(* Logix 5000 AddOnInstructionDefinition export SPEL_Above; software revision 30.01; part 2 of 9 *)

ADD_ON_INSTRUCTION SPEL_BaseGet   (* revision 1.0, vendor SEIKO EPSON CORP. *)
// Gets the base coordinate system.
VAR_INPUT
   Start : BOOL; {required}
END_VAR
VAR_OUTPUT
   InCycle : BOOL; {access Read Only, visible}
   Done : BOOL; {access Read Only, visible}
   Error : BOOL; {access Read Only, visible}
END_VAR
VAR_INPUT
   NumAxes : INT; {required}
END_VAR
VAR_OUTPUT
   BaseX : REAL; {visible}
   BaseY : REAL; {visible}
   BaseZ : REAL; {visible}
   BaseU : REAL; {visible}
   BaseV : REAL; {visible}
   BaseW : REAL; {visible}
END_VAR
VAR_IN_OUT
   ExtInputs : AB:ETHERNET_MODULE_INT_128Bytes:I:0; {required}
   ExtOutputs : AB:ETHERNET_MODULE_INT_128Bytes:O:0; {required}
END_VAR
VAR_OUTPUT
   ErrCode1 : INT; {access Read Only, visible}
   ErrCode2 : INT; {access Read Only, visible}
END_VAR
VAR
   Coordinatex1000 : DINT; {access None}
   Coordinate_INTS : INT[2]; {access None}
   OneShotStart : BOOL[32]; {access None}
   StartInit : BOOL[32]; {access None}
   ExecBaseGetW : SPEL_ExecCmd := (MaxTime := 3000); {access None}
   ExecBaseGetV : SPEL_ExecCmd := (MaxTime := 3000); {access None}
   ExecBaseGetU : SPEL_ExecCmd := (MaxTime := 3000); {access None}
   ExecBaseGetZ : SPEL_ExecCmd := (MaxTime := 3000); {access None}
   ExecBaseGetY : SPEL_ExecCmd := (MaxTime := 3000); {access None}
   ExecBaseGetX : SPEL_ExecCmd := (MaxTime := 3000); {access None}
   X6 : BOOL; {access None}
   ExecTimeout : DINT := 5000; {access None}
END_VAR

ROUTINE Logic   (* ladder *)
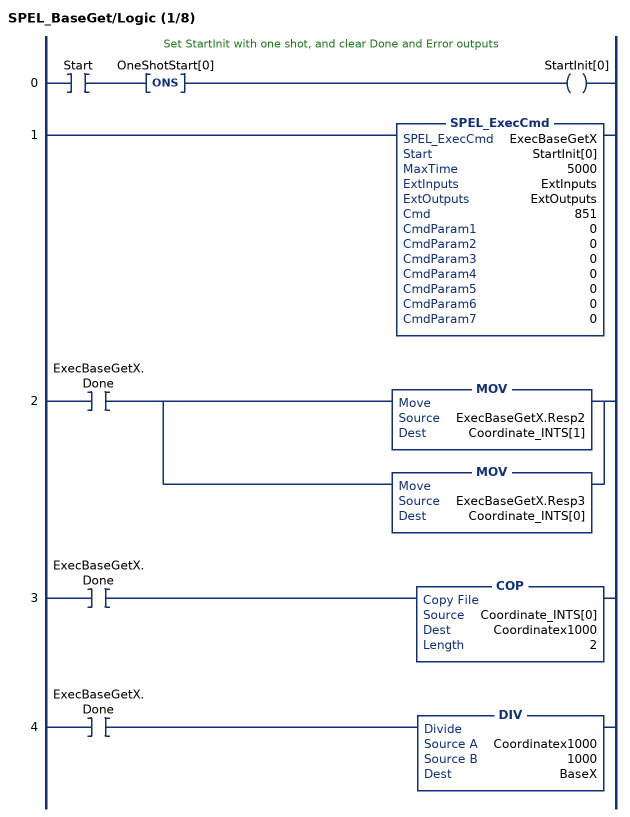
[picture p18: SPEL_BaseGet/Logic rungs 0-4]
   // Set StartInit with one shot, and clear Done and Error outputs
   0: XIC(Start)ONS(OneShotStart[0])OTE(StartInit[0]);
   1: SPEL_ExecCmd(ExecBaseGetX,StartInit[0],5000,ExtInputs,ExtOutputs,851,0,0,0,0,0,0,0);
   2: XIC(ExecBaseGetX.Done)[MOV(ExecBaseGetX.Resp2,Coordinate_INTS[1]) ,MOV(ExecBaseGetX.Resp3,Coordinate_INTS[0]) ];
   3: XIC(ExecBaseGetX.Done)COP(Coordinate_INTS[0],Coordinatex1000,2);
   4: XIC(ExecBaseGetX.Done)DIV(Coordinatex1000,1000,BaseX);
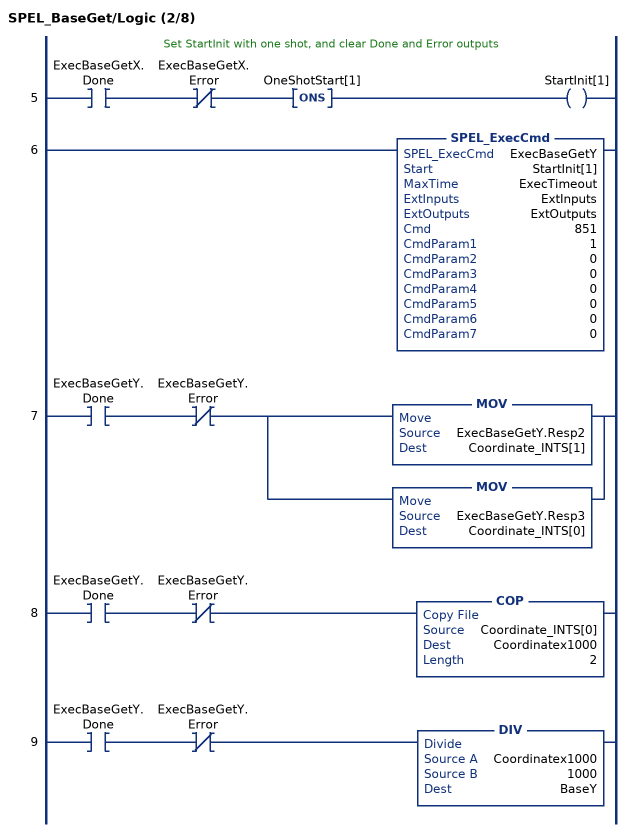
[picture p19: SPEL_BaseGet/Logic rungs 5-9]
   // Set StartInit with one shot, and clear Done and Error outputs
   5: XIC(ExecBaseGetX.Done)XIO(ExecBaseGetX.Error)ONS(OneShotStart[1])OTE(StartInit[1]);
   6: SPEL_ExecCmd(ExecBaseGetY,StartInit[1],ExecTimeout,ExtInputs,ExtOutputs,851,1,0,0,0,0,0,0);
   7: XIC(ExecBaseGetY.Done)XIO(ExecBaseGetY.Error)[MOV(ExecBaseGetY.Resp2,Coordinate_INTS[1]) ,MOV(ExecBaseGetY.Resp3,Coordinate_INTS[0]) ];
   8: XIC(ExecBaseGetY.Done)XIO(ExecBaseGetY.Error)COP(Coordinate_INTS[0],Coordinatex1000,2);
   9: XIC(ExecBaseGetY.Done)XIO(ExecBaseGetY.Error)DIV(Coordinatex1000,1000,BaseY);
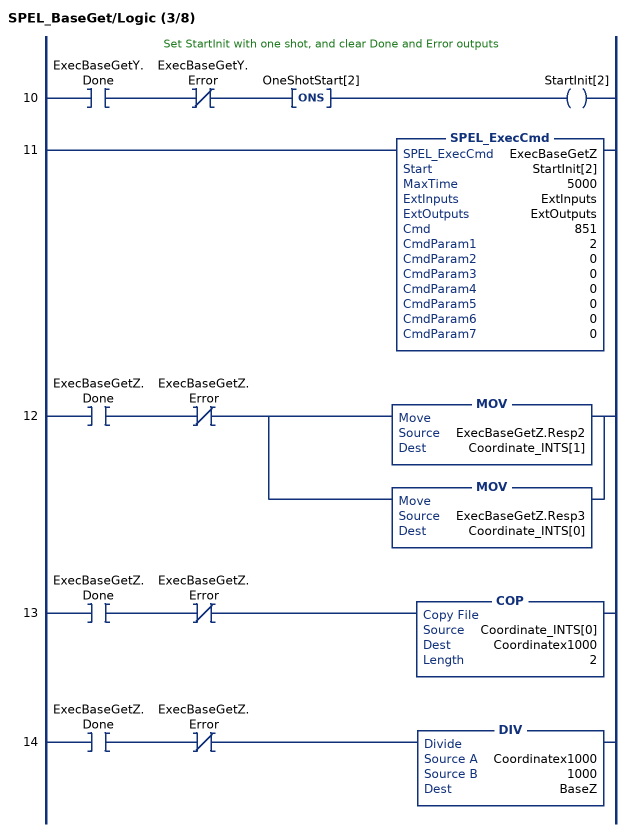
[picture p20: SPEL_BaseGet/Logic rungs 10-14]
   // Set StartInit with one shot, and clear Done and Error outputs
   10: XIC(ExecBaseGetY.Done)XIO(ExecBaseGetY.Error)ONS(OneShotStart[2])OTE(StartInit[2]);
   11: SPEL_ExecCmd(ExecBaseGetZ,StartInit[2],5000,ExtInputs,ExtOutputs,851,2,0,0,0,0,0,0);
   12: XIC(ExecBaseGetZ.Done)XIO(ExecBaseGetZ.Error)[MOV(ExecBaseGetZ.Resp2,Coordinate_INTS[1]) ,MOV(ExecBaseGetZ.Resp3,Coordinate_INTS[0]) ];
   13: XIC(ExecBaseGetZ.Done)XIO(ExecBaseGetZ.Error)COP(Coordinate_INTS[0],Coordinatex1000,2);
   14: XIC(ExecBaseGetZ.Done)XIO(ExecBaseGetZ.Error)DIV(Coordinatex1000,1000,BaseZ);
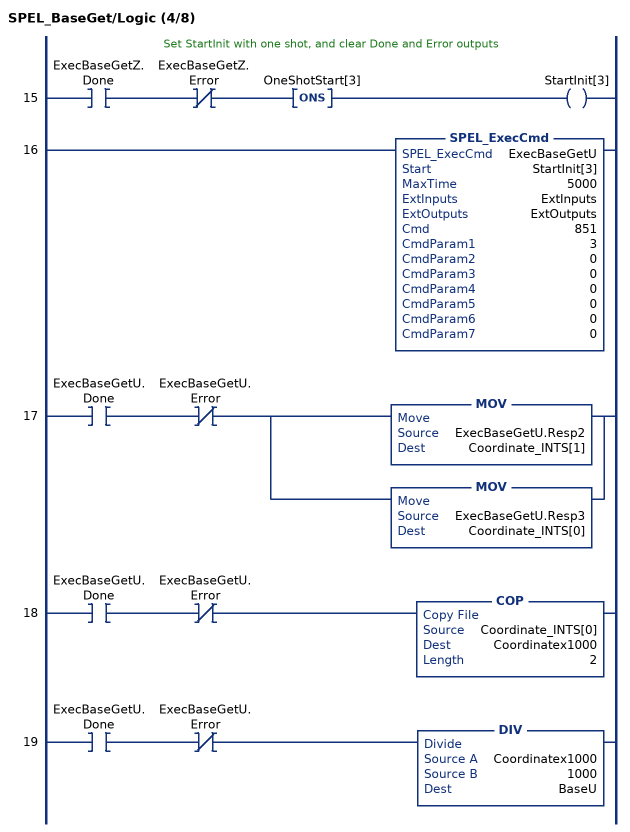
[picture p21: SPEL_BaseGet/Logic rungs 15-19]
   // Set StartInit with one shot, and clear Done and Error outputs
   15: XIC(ExecBaseGetZ.Done)XIO(ExecBaseGetZ.Error)ONS(OneShotStart[3])OTE(StartInit[3]);
   16: SPEL_ExecCmd(ExecBaseGetU,StartInit[3],5000,ExtInputs,ExtOutputs,851,3,0,0,0,0,0,0);
   17: XIC(ExecBaseGetU.Done)XIO(ExecBaseGetU.Error)[MOV(ExecBaseGetU.Resp2,Coordinate_INTS[1]) ,MOV(ExecBaseGetU.Resp3,Coordinate_INTS[0]) ];
   18: XIC(ExecBaseGetU.Done)XIO(ExecBaseGetU.Error)COP(Coordinate_INTS[0],Coordinatex1000,2);
   19: XIC(ExecBaseGetU.Done)XIO(ExecBaseGetU.Error)DIV(Coordinatex1000,1000,BaseU);
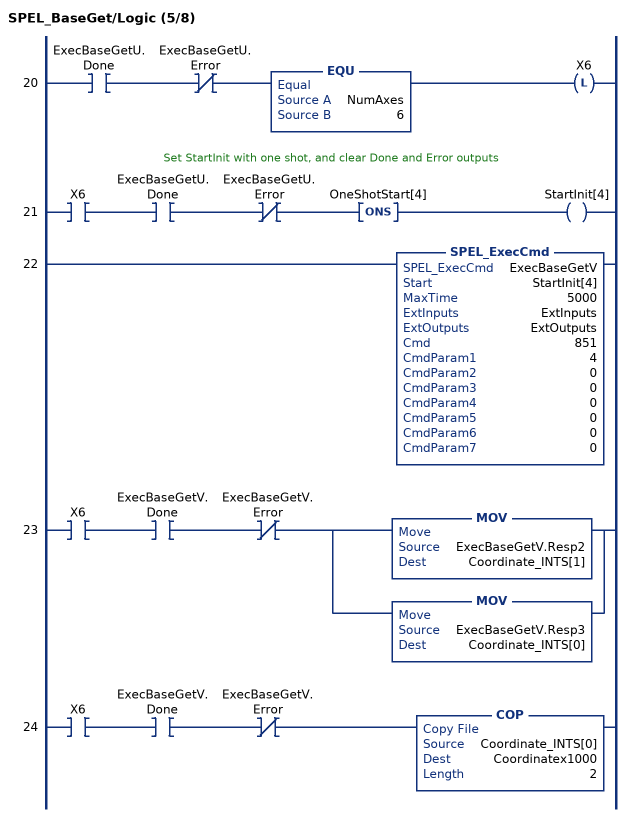
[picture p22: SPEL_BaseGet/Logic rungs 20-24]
   20: XIC(ExecBaseGetU.Done)XIO(ExecBaseGetU.Error)EQU(NumAxes,6)OTL(X6);
   // Set StartInit with one shot, and clear Done and Error outputs
   21: XIC(X6)XIC(ExecBaseGetU.Done)XIO(ExecBaseGetU.Error)ONS(OneShotStart[4])OTE(StartInit[4]);
   22: SPEL_ExecCmd(ExecBaseGetV,StartInit[4],5000,ExtInputs,ExtOutputs,851,4,0,0,0,0,0,0);
   23: XIC(X6)XIC(ExecBaseGetV.Done)XIO(ExecBaseGetV.Error)[MOV(ExecBaseGetV.Resp2,Coordinate_INTS[1]) ,MOV(ExecBaseGetV.Resp3,Coordinate_INTS[0]) ];
   24: XIC(X6)XIC(ExecBaseGetV.Done)XIO(ExecBaseGetV.Error)COP(Coordinate_INTS[0],Coordinatex1000,2);
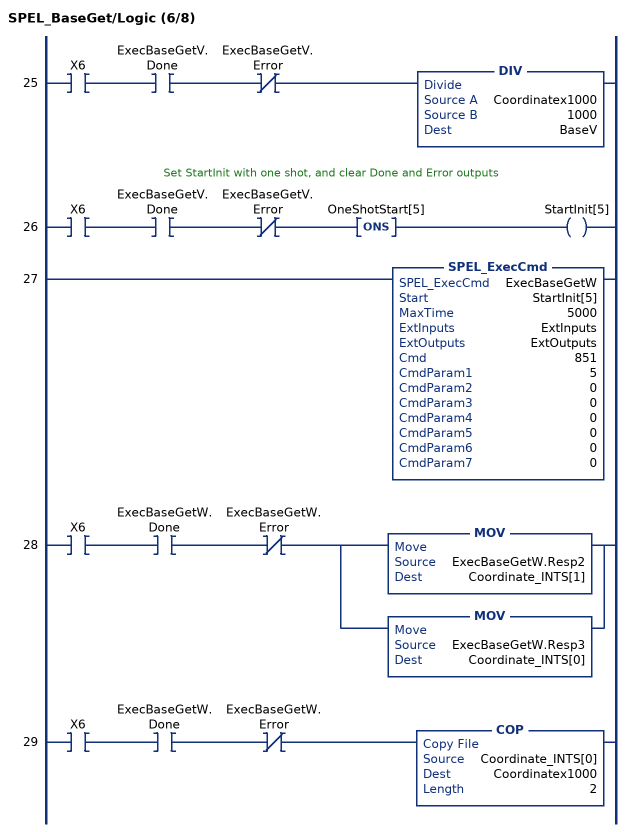
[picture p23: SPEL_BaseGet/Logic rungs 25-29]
   25: XIC(X6)XIC(ExecBaseGetV.Done)XIO(ExecBaseGetV.Error)DIV(Coordinatex1000,1000,BaseV);
   // Set StartInit with one shot, and clear Done and Error outputs
   26: XIC(X6)XIC(ExecBaseGetV.Done)XIO(ExecBaseGetV.Error)ONS(OneShotStart[5])OTE(StartInit[5]);
   27: SPEL_ExecCmd(ExecBaseGetW,StartInit[5],5000,ExtInputs,ExtOutputs,851,5,0,0,0,0,0,0);
   28: XIC(X6)XIC(ExecBaseGetW.Done)XIO(ExecBaseGetW.Error)[MOV(ExecBaseGetW.Resp2,Coordinate_INTS[1]) ,MOV(ExecBaseGetW.Resp3,Coordinate_INTS[0]) ];
   29: XIC(X6)XIC(ExecBaseGetW.Done)XIO(ExecBaseGetW.Error)COP(Coordinate_INTS[0],Coordinatex1000,2);
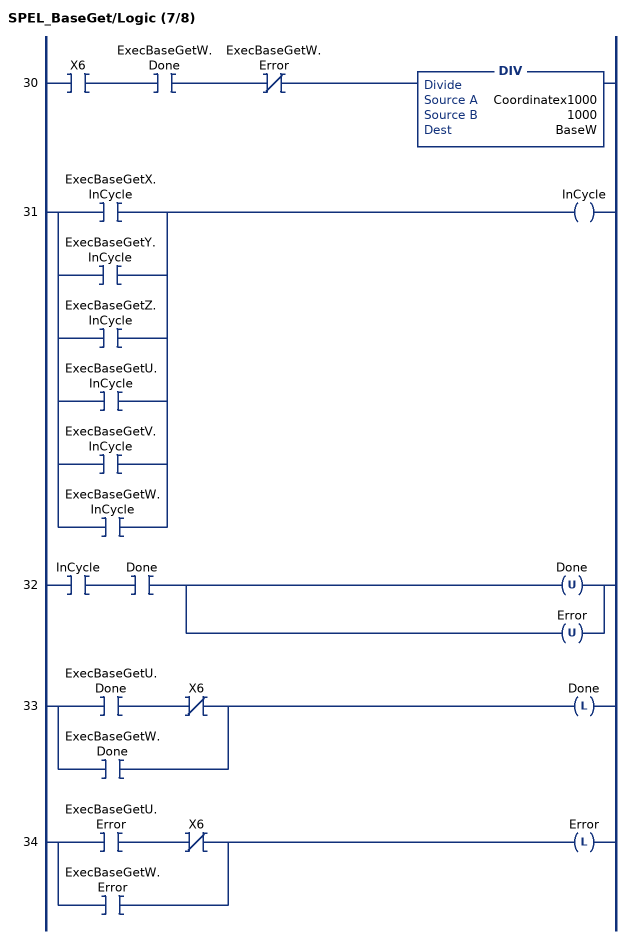
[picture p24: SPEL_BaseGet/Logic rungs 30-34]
   30: XIC(X6)XIC(ExecBaseGetW.Done)XIO(ExecBaseGetW.Error)DIV(Coordinatex1000,1000,BaseW);
   31: [XIC(ExecBaseGetX.InCycle) ,XIC(ExecBaseGetY.InCycle) ,XIC(ExecBaseGetZ.InCycle) ,XIC(ExecBaseGetU.InCycle) ,XIC(ExecBaseGetV.InCycle) ,XIC(ExecBaseGetW.InCycle) ]OTE(InCycle);
   32: XIC(InCycle)XIC(Done)[OTU(Done) ,OTU(Error) ];
   33: [XIC(ExecBaseGetU.Done) XIO(X6) ,XIC(ExecBaseGetW.Done) ]OTL(Done);
   34: [XIC(ExecBaseGetU.Error) XIO(X6) ,XIC(ExecBaseGetW.Error) ]OTL(Error);
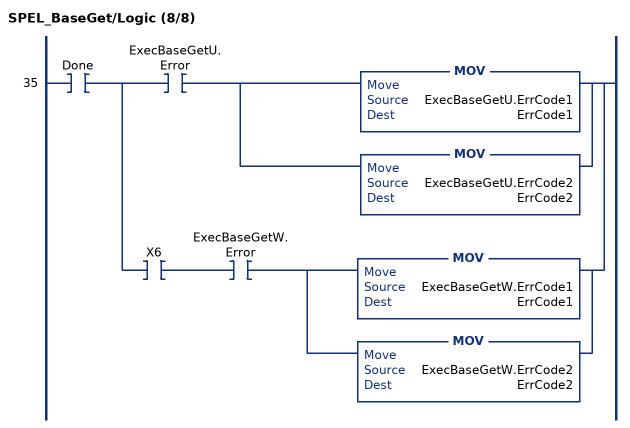
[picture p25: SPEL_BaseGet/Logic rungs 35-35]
   35: XIC(Done)[XIC(ExecBaseGetU.Error) [MOV(ExecBaseGetU.ErrCode1,ErrCode1) ,MOV(ExecBaseGetU.ErrCode2,ErrCode2) ] ,XIC(X6) XIC(ExecBaseGetW.Error) [MOV(ExecBaseGetW.ErrCode1,ErrCode1) ,MOV(ExecBaseGetW.ErrCode2,ErrCode2) ] ];
END_ROUTINE
END_ADD_ON_INSTRUCTION

ADD_ON_INSTRUCTION SPEL_BaseSet   (* revision 1.0, vendor SEIKO EPSON CORP. *)
// Sets the base coordinate system.
VAR_OUTPUT
   InCycle : BOOL; {access Read Only, visible}
   Done : BOOL; {access Read Only, visible}
END_VAR
VAR_INPUT
   Start : BOOL; {required}
END_VAR
VAR_OUTPUT
   Error : BOOL; {access Read Only, visible}
END_VAR
VAR_INPUT
   NumAxes : INT; {required}
   BaseX : REAL; {required}
   BaseY : REAL; {required}
   BaseZ : REAL; {required}
   BaseU : REAL; {required}
   BaseV : REAL; {required}
   BaseW : REAL; {required}
END_VAR
VAR_IN_OUT
   ExtInputs : AB:ETHERNET_MODULE_INT_128Bytes:I:0; {required}
   ExtOutputs : AB:ETHERNET_MODULE_INT_128Bytes:O:0; {required}
END_VAR
VAR_OUTPUT
   ErrCode1 : INT; {access Read Only, visible}
   ErrCode2 : INT; {access Read Only, visible}
END_VAR
VAR
   Valuex1000 : DINT; {access None}
   Value_INTS : INT[2]; {access None}
   StartInit : BOOL[32]; {access None}
   OneShotStart : BOOL[32]; {access None}
   ExecBaseSetX : SPEL_ExecCmd := (MaxTime := 3000); {access None}
   ExecBaseSetW : SPEL_ExecCmd := (MaxTime := 3000); {access None}
   ExecBaseSetV : SPEL_ExecCmd := (MaxTime := 3000); {access None}
   ExecBaseSetU : SPEL_ExecCmd := (MaxTime := 3000); {access None}
   ExecBaseSetZ : SPEL_ExecCmd := (MaxTime := 3000); {access None}
   ExecBaseSetY : SPEL_ExecCmd := (MaxTime := 3000); {access None}
   X6 : BOOL; {access None}
   ExecTimeout : DINT; {access None}
END_VAR

ROUTINE Logic   (* ladder *)
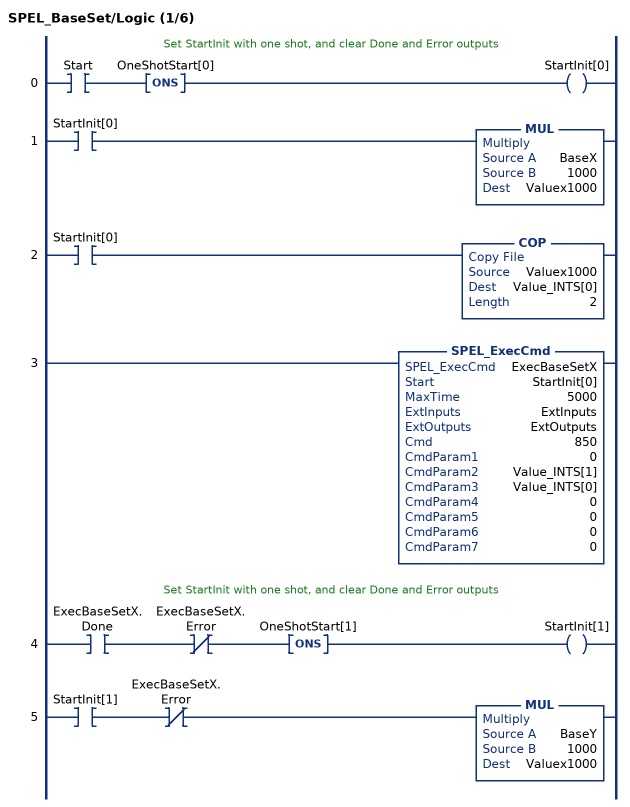
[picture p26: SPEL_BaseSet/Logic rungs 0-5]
   // Set StartInit with one shot, and clear Done and Error outputs
   0: XIC(Start)ONS(OneShotStart[0])OTE(StartInit[0]);
   1: XIC(StartInit[0])MUL(BaseX,1000,Valuex1000);
   2: XIC(StartInit[0])COP(Valuex1000,Value_INTS[0],2);
   3: SPEL_ExecCmd(ExecBaseSetX,StartInit[0],5000,ExtInputs,ExtOutputs,850,0,Value_INTS[1],Value_INTS[0],0,0,0,0);
   // Set StartInit with one shot, and clear Done and Error outputs
   4: XIC(ExecBaseSetX.Done)XIO(ExecBaseSetX.Error)ONS(OneShotStart[1])OTE(StartInit[1]);
   5: XIC(StartInit[1])XIO(ExecBaseSetX.Error)MUL(BaseY,1000,Valuex1000);
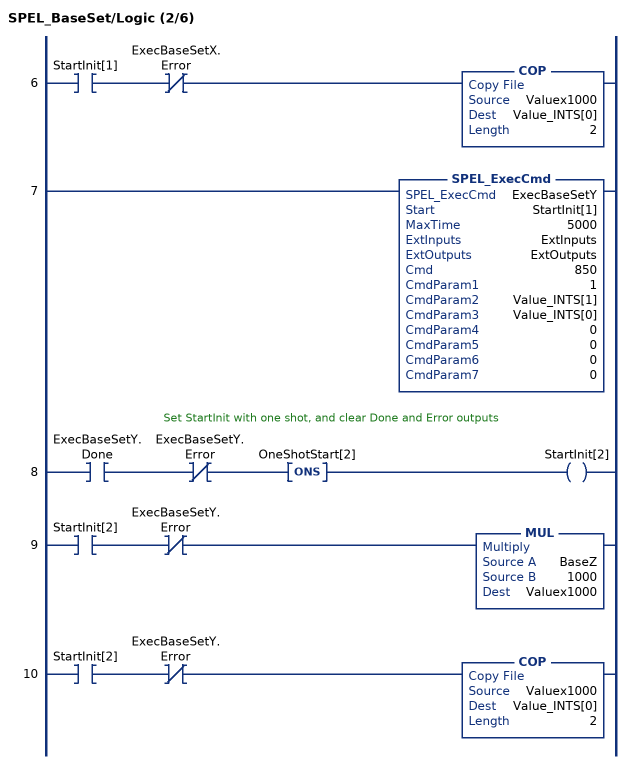
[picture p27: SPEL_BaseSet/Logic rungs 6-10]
   6: XIC(StartInit[1])XIO(ExecBaseSetX.Error)COP(Valuex1000,Value_INTS[0],2);
   7: SPEL_ExecCmd(ExecBaseSetY,StartInit[1],5000,ExtInputs,ExtOutputs,850,1,Value_INTS[1],Value_INTS[0],0,0,0,0);
   // Set StartInit with one shot, and clear Done and Error outputs
   8: XIC(ExecBaseSetY.Done)XIO(ExecBaseSetY.Error)ONS(OneShotStart[2])OTE(StartInit[2]);
   9: XIC(StartInit[2])XIO(ExecBaseSetY.Error)MUL(BaseZ,1000,Valuex1000);
   10: XIC(StartInit[2])XIO(ExecBaseSetY.Error)COP(Valuex1000,Value_INTS[0],2);
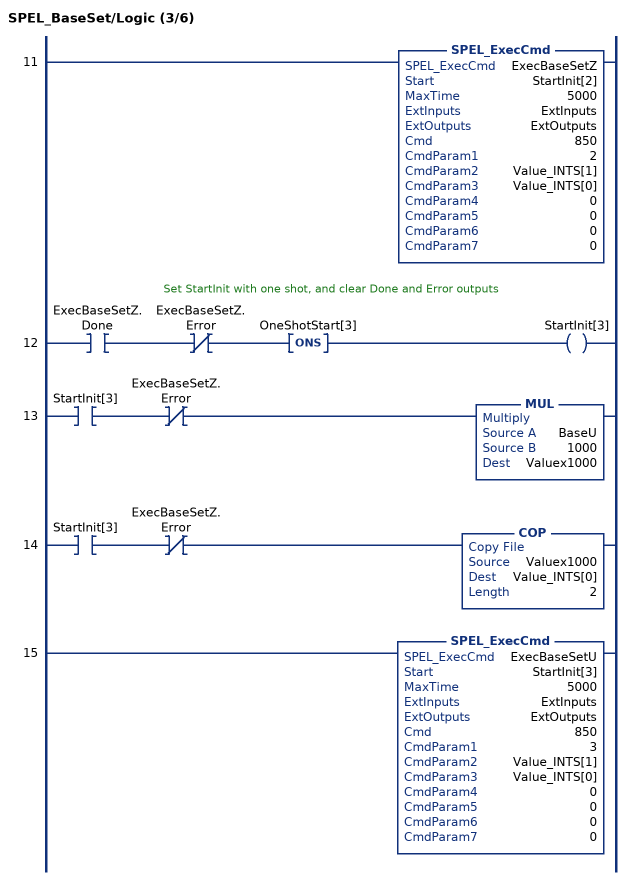
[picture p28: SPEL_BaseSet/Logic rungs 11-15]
   11: SPEL_ExecCmd(ExecBaseSetZ,StartInit[2],5000,ExtInputs,ExtOutputs,850,2,Value_INTS[1],Value_INTS[0],0,0,0,0);
   // Set StartInit with one shot, and clear Done and Error outputs
   12: XIC(ExecBaseSetZ.Done)XIO(ExecBaseSetZ.Error)ONS(OneShotStart[3])OTE(StartInit[3]);
   13: XIC(StartInit[3])XIO(ExecBaseSetZ.Error)MUL(BaseU,1000,Valuex1000);
   14: XIC(StartInit[3])XIO(ExecBaseSetZ.Error)COP(Valuex1000,Value_INTS[0],2);
   15: SPEL_ExecCmd(ExecBaseSetU,StartInit[3],5000,ExtInputs,ExtOutputs,850,3,Value_INTS[1],Value_INTS[0],0,0,0,0);
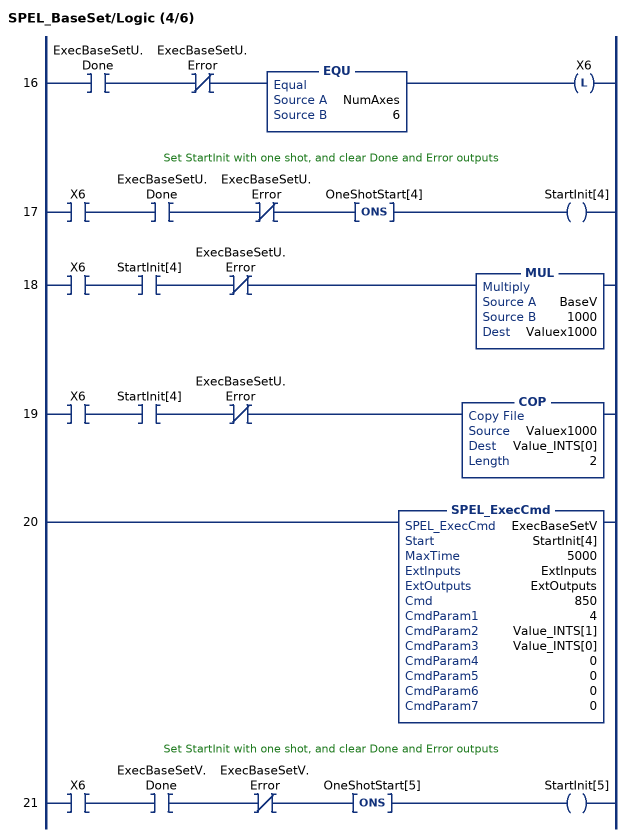
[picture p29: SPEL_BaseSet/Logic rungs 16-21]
   16: XIC(ExecBaseSetU.Done)XIO(ExecBaseSetU.Error)EQU(NumAxes,6)OTL(X6);
   // Set StartInit with one shot, and clear Done and Error outputs
   17: XIC(X6)XIC(ExecBaseSetU.Done)XIO(ExecBaseSetU.Error)ONS(OneShotStart[4])OTE(StartInit[4]);
   18: XIC(X6)XIC(StartInit[4])XIO(ExecBaseSetU.Error)MUL(BaseV,1000,Valuex1000);
   19: XIC(X6)XIC(StartInit[4])XIO(ExecBaseSetU.Error)COP(Valuex1000,Value_INTS[0],2);
   20: SPEL_ExecCmd(ExecBaseSetV,StartInit[4],5000,ExtInputs,ExtOutputs,850,4,Value_INTS[1],Value_INTS[0],0,0,0,0);
   // Set StartInit with one shot, and clear Done and Error outputs
   21: XIC(X6)XIC(ExecBaseSetV.Done)XIO(ExecBaseSetV.Error)ONS(OneShotStart[5])OTE(StartInit[5]);
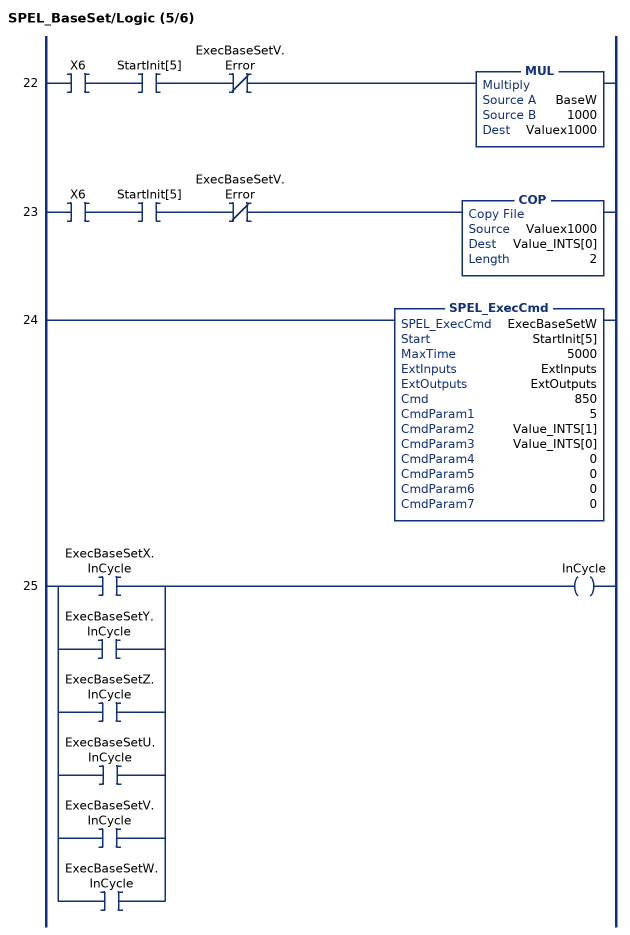
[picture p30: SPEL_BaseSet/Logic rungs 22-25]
   22: XIC(X6)XIC(StartInit[5])XIO(ExecBaseSetV.Error)MUL(BaseW,1000,Valuex1000);
   23: XIC(X6)XIC(StartInit[5])XIO(ExecBaseSetV.Error)COP(Valuex1000,Value_INTS[0],2);
   24: SPEL_ExecCmd(ExecBaseSetW,StartInit[5],5000,ExtInputs,ExtOutputs,850,5,Value_INTS[1],Value_INTS[0],0,0,0,0);
   25: [XIC(ExecBaseSetX.InCycle) ,XIC(ExecBaseSetY.InCycle) ,XIC(ExecBaseSetZ.InCycle) ,XIC(ExecBaseSetU.InCycle) ,XIC(ExecBaseSetV.InCycle) ,XIC(ExecBaseSetW.InCycle) ]OTE(InCycle);
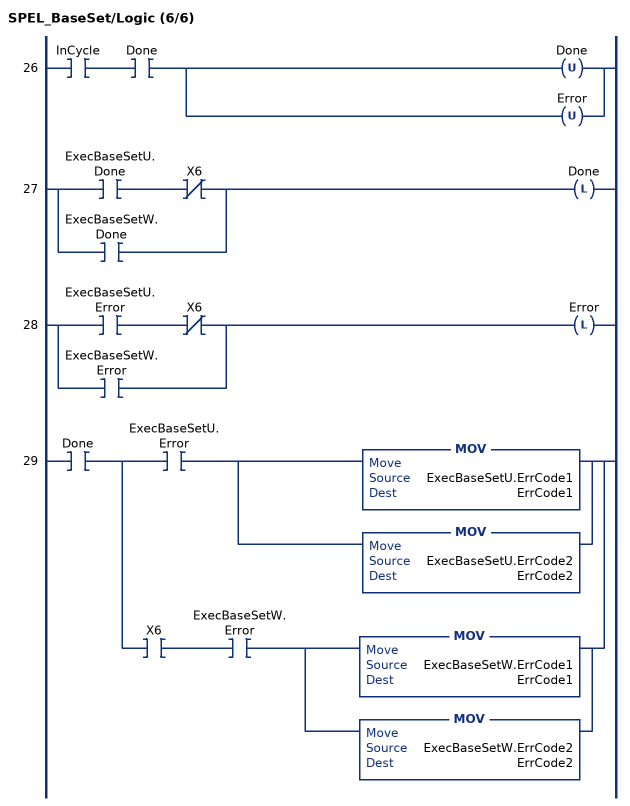
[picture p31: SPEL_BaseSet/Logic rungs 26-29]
   26: XIC(InCycle)XIC(Done)[OTU(Done) ,OTU(Error) ];
   27: [XIC(ExecBaseSetU.Done) XIO(X6) ,XIC(ExecBaseSetW.Done) ]OTL(Done);
   28: [XIC(ExecBaseSetU.Error) XIO(X6) ,XIC(ExecBaseSetW.Error) ]OTL(Error);
   29: XIC(Done)[XIC(ExecBaseSetU.Error) [MOV(ExecBaseSetU.ErrCode1,ErrCode1) ,MOV(ExecBaseSetU.ErrCode2,ErrCode2) ] ,XIC(X6) XIC(ExecBaseSetW.Error) [MOV(ExecBaseSetW.ErrCode1,ErrCode1) ,MOV(ExecBaseSetW.ErrCode2,ErrCode2) ] ];
END_ROUTINE
END_ADD_ON_INSTRUCTION

ADD_ON_INSTRUCTION SPEL_Below   (* revision 1.0, vendor SEIKO EPSON CORP. *)
// Sets the elbow orientation of the specified point to Below.
VAR_INPUT
   Start : BOOL; {required}
END_VAR
VAR_OUTPUT
   InCycle : BOOL; {access Read Only, visible}
   Done : BOOL; {access Read Only, visible}
   Error : BOOL; {access Read Only, visible}
END_VAR
VAR_INPUT
   Point : INT; {required}
END_VAR
VAR_IN_OUT
   ExtInputs : AB:ETHERNET_MODULE_INT_128Bytes:I:0; {required}
   ExtOutputs : AB:ETHERNET_MODULE_INT_128Bytes:O:0; {required}
END_VAR
VAR_OUTPUT
   ErrCode1 : INT; {access Read Only, visible}
   ErrCode2 : INT; {access Read Only, visible}
END_VAR
VAR
   ExecBelow : SPEL_ExecCmd := (MaxTime := 3000); {access None}
   OneShotStart : BOOL; {access None}
   StartCoil : BOOL; {access None}
   ExecTimeout : DINT; {access None}
END_VAR

ROUTINE Logic   (* ladder *)
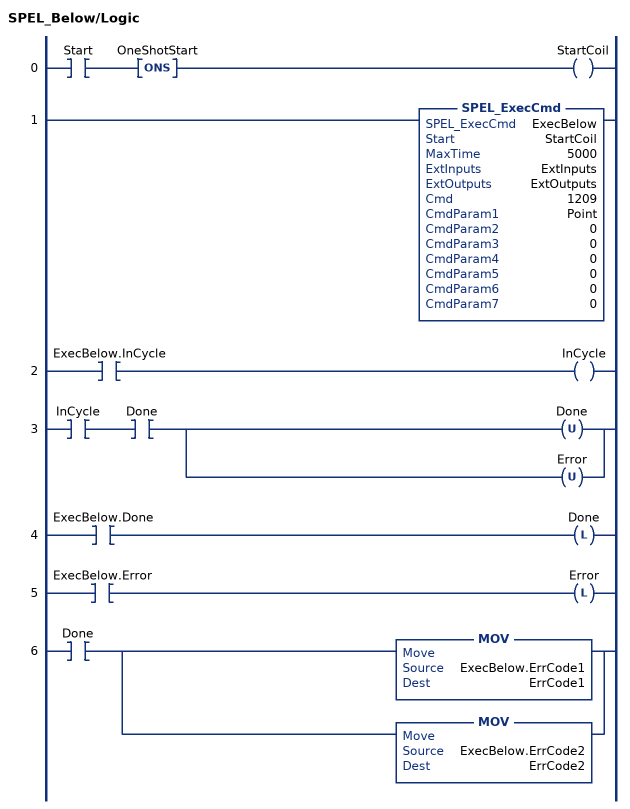
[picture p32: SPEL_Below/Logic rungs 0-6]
   0: XIC(Start)ONS(OneShotStart)OTE(StartCoil);
   1: SPEL_ExecCmd(ExecBelow,StartCoil,5000,ExtInputs,ExtOutputs,1209,Point,0,0,0,0,0,0);
   2: XIC(ExecBelow.InCycle)OTE(InCycle);
   3: XIC(InCycle)XIC(Done)[OTU(Done) ,OTU(Error) ];
   4: XIC(ExecBelow.Done)OTL(Done);
   5: XIC(ExecBelow.Error)OTL(Error);
   6: XIC(Done)[MOV(ExecBelow.ErrCode1,ErrCode1) ,MOV(ExecBelow.ErrCode2,ErrCode2) ];
END_ROUTINE
END_ADD_ON_INSTRUCTION

ADD_ON_INSTRUCTION SPEL_CPOff   (* revision 1.0, vendor SEIKO EPSON CORP. *)
// Turns off Continuous Path.
VAR_INPUT
   Start : BOOL; {access Read Only, required}
END_VAR
VAR_OUTPUT
   InCycle : BOOL; {access Read Only, visible}
   Done : BOOL; {access Read Only, visible}
   Error : BOOL; {access Read Only, visible}
END_VAR
VAR_IN_OUT
   ExtInputs : AB:ETHERNET_MODULE_INT_128Bytes:I:0; {required}
   ExtOutputs : AB:ETHERNET_MODULE_INT_128Bytes:O:0; {required}
END_VAR
VAR_OUTPUT
   ErrCode1 : INT; {access Read Only, visible}
   ErrCode2 : INT; {access Read Only, visible}
END_VAR
VAR
   ExecCPOff : SPEL_ExecCmd := (MaxTime := 3000); {access None}
        .INCYCLE   // ExecInCycle
        .DONE   // ExecDone
        .ERROR   // ExecError
   OneShotStart : BOOL; {access None}
   StartCoil : BOOL; {access None}
   ExecTimeout : DINT; {access None}
END_VAR

ROUTINE Logic   (* ladder *)
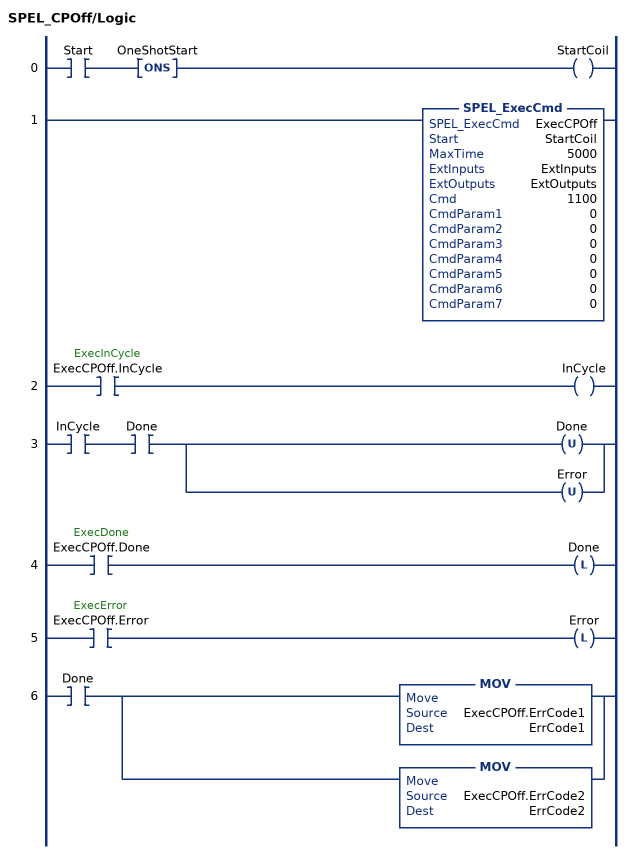
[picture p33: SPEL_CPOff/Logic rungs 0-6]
   0: XIC(Start)ONS(OneShotStart)OTE(StartCoil);
   1: SPEL_ExecCmd(ExecCPOff,StartCoil,5000,ExtInputs,ExtOutputs,1100,0,0,0,0,0,0,0);
   2: XIC(ExecCPOff.InCycle)OTE(InCycle);
   3: XIC(InCycle)XIC(Done)[OTU(Done) ,OTU(Error) ];
   4: XIC(ExecCPOff.Done)OTL(Done);
   5: XIC(ExecCPOff.Error)OTL(Error);
   6: XIC(Done)[MOV(ExecCPOff.ErrCode1,ErrCode1) ,MOV(ExecCPOff.ErrCode2,ErrCode2) ];
END_ROUTINE
END_ADD_ON_INSTRUCTION

ADD_ON_INSTRUCTION SPEL_CPOn   (* revision 1.0, vendor SEIKO EPSON CORP. *)
// Turns on Continuous Path.
VAR_INPUT
   Start : BOOL; {access Read Only, required}
END_VAR
VAR_OUTPUT
   InCycle : BOOL; {access Read Only, visible}
   Done : BOOL; {access Read Only, visible}
   Error : BOOL; {access Read Only, visible}
END_VAR
VAR_IN_OUT
   ExtInputs : AB:ETHERNET_MODULE_INT_128Bytes:I:0; {required}
   ExtOutputs : AB:ETHERNET_MODULE_INT_128Bytes:O:0; {required}
END_VAR
VAR_OUTPUT
   ErrCode1 : INT; {access Read Only, visible}
   ErrCode2 : INT; {access Read Only, visible}
END_VAR
VAR
   ExecCPOn : SPEL_ExecCmd := (MaxTime := 3000); {access None}
        .INCYCLE   // ExecInCycle
        .DONE   // ExecDone
        .ERROR   // ExecError
   OneShotStart : BOOL; {access None}
   StartCoil : BOOL; {access None}
   ExecTimeout : DINT; {access None}
END_VAR

ROUTINE Logic   (* ladder *)
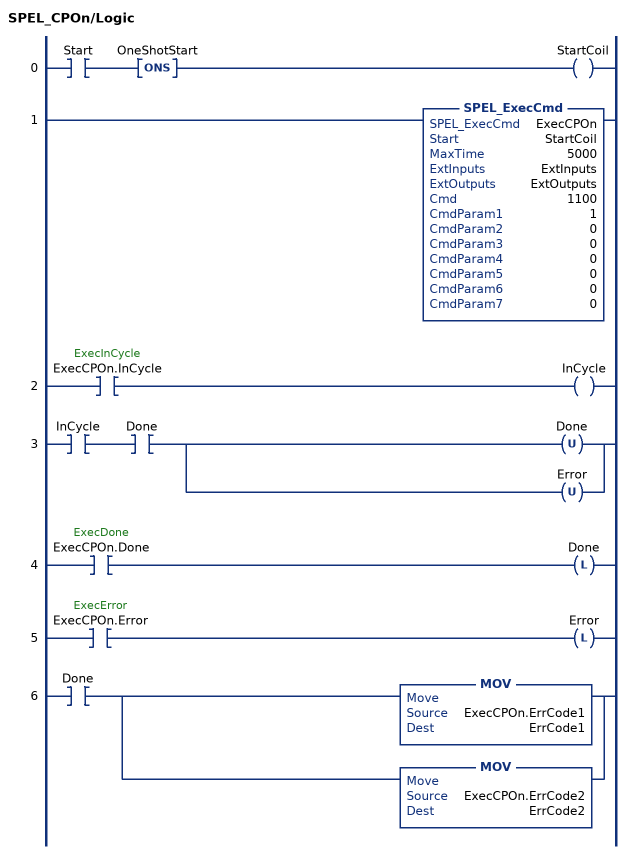
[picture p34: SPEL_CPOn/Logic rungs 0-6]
   0: XIC(Start)ONS(OneShotStart)OTE(StartCoil);
   1: SPEL_ExecCmd(ExecCPOn,StartCoil,5000,ExtInputs,ExtOutputs,1100,1,0,0,0,0,0,0);
   2: XIC(ExecCPOn.InCycle)OTE(InCycle);
   3: XIC(InCycle)XIC(Done)[OTU(Done) ,OTU(Error) ];
   4: XIC(ExecCPOn.Done)OTL(Done);
   5: XIC(ExecCPOn.Error)OTL(Error);
   6: XIC(Done)[MOV(ExecCPOn.ErrCode1,ErrCode1) ,MOV(ExecCPOn.ErrCode2,ErrCode2) ];
END_ROUTINE
END_ADD_ON_INSTRUCTION

ADD_ON_INSTRUCTION SPEL_FineGet   (* revision 1.0, vendor SEIKO EPSON CORP. *)
// Gets the positioning end judgement range for all joints.
VAR_INPUT
   Start : BOOL; {required}
END_VAR
VAR_OUTPUT
   InCycle : BOOL; {access Read Only, visible}
   Done : BOOL; {access Read Only, visible}
   Error : BOOL; {access Read Only, visible}
   Axis1 : DINT; {visible}
   Axis2 : DINT; {visible}
   Axis3 : DINT; {visible}
   Axis4 : DINT; {visible}
   Axis5 : DINT; {visible}
   Axis6 : DINT; {visible}
END_VAR
VAR_IN_OUT
   ExtInputs : AB:ETHERNET_MODULE_INT_128Bytes:I:0; {required}
   ExtOutputs : AB:ETHERNET_MODULE_INT_128Bytes:O:0; {required}
END_VAR
VAR_OUTPUT
   ErrCode1 : INT; {access Read Only, visible}
   ErrCode2 : INT; {access Read Only, visible}
END_VAR
VAR
   ExecFineGet : SPEL_ExecCmd := (MaxTime := 3000); {access None}
   OneShotStart : BOOL; {access None}
   StartCoil : BOOL; {access None}
   ExecTimeout : DINT; {access None}
END_VAR

ROUTINE Logic   (* ladder *)
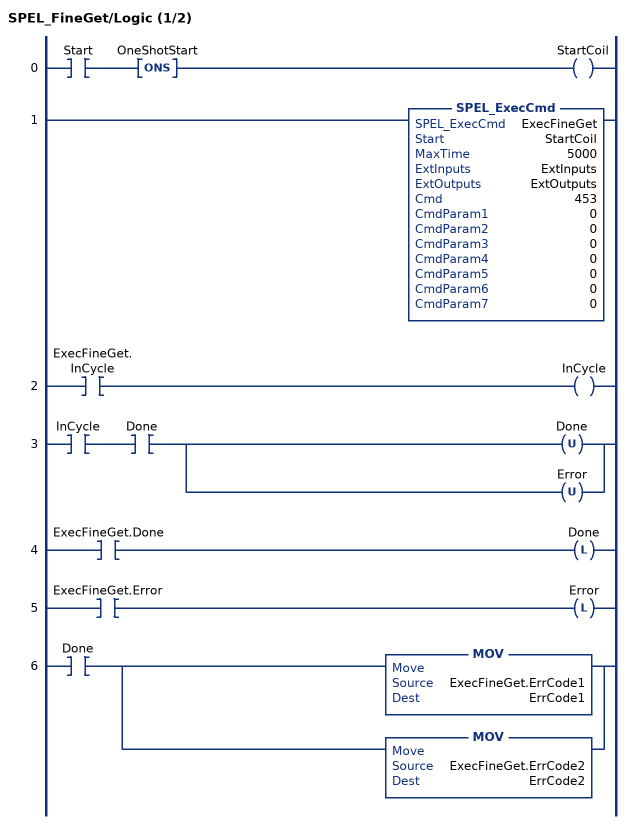
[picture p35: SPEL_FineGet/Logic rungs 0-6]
   0: XIC(Start)ONS(OneShotStart)OTE(StartCoil);
   1: SPEL_ExecCmd(ExecFineGet,StartCoil,5000,ExtInputs,ExtOutputs,453,0,0,0,0,0,0,0);
   2: XIC(ExecFineGet.InCycle)OTE(InCycle);
   3: XIC(InCycle)XIC(Done)[OTU(Done) ,OTU(Error) ];
   4: XIC(ExecFineGet.Done)OTL(Done);
   5: XIC(ExecFineGet.Error)OTL(Error);
   6: XIC(Done)[MOV(ExecFineGet.ErrCode1,ErrCode1) ,MOV(ExecFineGet.ErrCode2,ErrCode2) ];
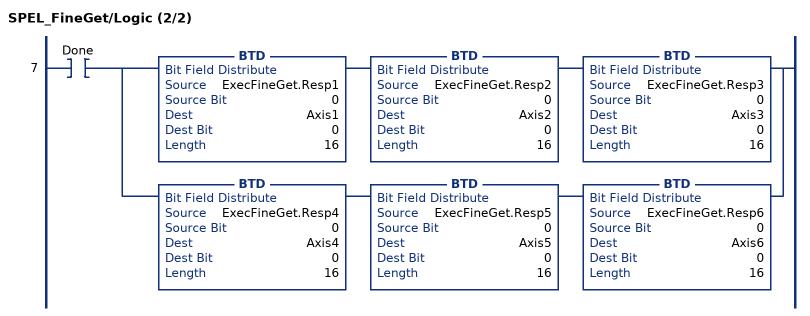
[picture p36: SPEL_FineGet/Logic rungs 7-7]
   7: XIC(Done)[BTD(ExecFineGet.Resp1,0,Axis1,0,16) BTD(ExecFineGet.Resp2,0,Axis2,0,16) BTD(ExecFineGet.Resp3,0,Axis3,0,16) ,BTD(ExecFineGet.Resp4,0,Axis4,0,16) BTD(ExecFineGet.Resp5,0,Axis5,0,16) BTD(ExecFineGet.Resp6,0,Axis6,0,16) ];
END_ROUTINE
END_ADD_ON_INSTRUCTION
